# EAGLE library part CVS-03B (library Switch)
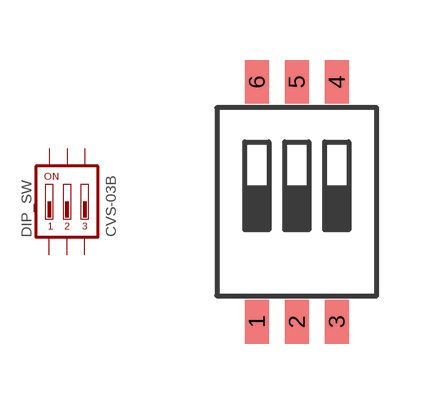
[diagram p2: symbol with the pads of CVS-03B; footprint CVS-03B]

Designator prefix DIP_SW

## CVS-03B  [CVS-03B]
1  1  pas
2  2  pas
3  3  pas
4  4  pas
5  5  pas
6  6  pas

## Footprint CVS-03B (pad centres in mm)
smd 0.6 x 1.1: 1 -1,-3; 2 0,-3; 3 1,-3; 4 1,3; 5 0,3; 6 -1,3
